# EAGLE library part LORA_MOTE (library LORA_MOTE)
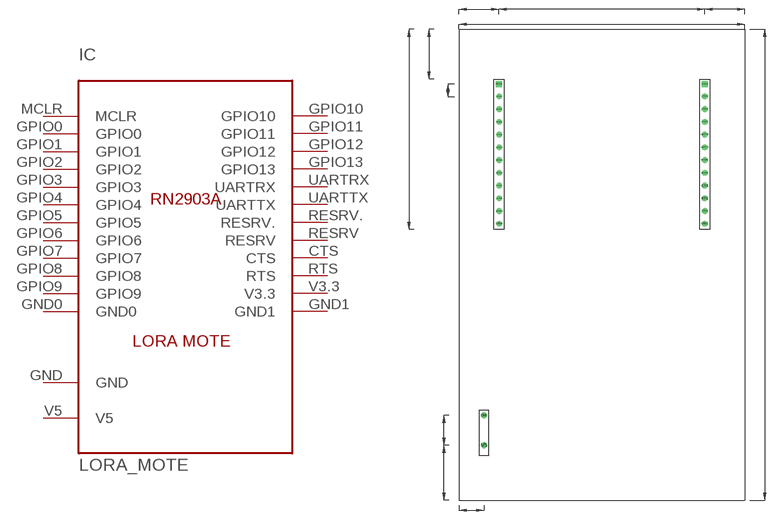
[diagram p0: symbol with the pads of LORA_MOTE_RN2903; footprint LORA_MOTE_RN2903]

Designator prefix IC

## LORA_MOTE  [LORA_MOTE_RN2903]
CTS  CTS
GND  GND
GND0  GND0
GND1  GND1
GPIO0  GPIO0
GPIO1  GPIO1
GPIO2  GPIO2
GPIO3  GPIO3
GPIO4  GPIO4
GPIO5  GPIO5
GPIO6  GPIO6
GPIO7  GPIO7
GPIO8  GPIO8
GPIO9  GPIO9
GPIO10  GPIO10
GPIO11  GPIO11
GPIO12  GPIO12
GPIO13  GPIO13
MCLR  MCLR
RESRV  RESRV
RESRV.  RESRV.
RTS  RTS
UARTRX  UARTRX
UARTTX  UARTTX
V3.3  V3.3
V5  V5

## Footprint LORA_MOTE_RN2903 (pad centres in mm)
drill 0.65: CTS 20.03,8.79; GND -24,-37; GND0 -20.97,1.17; GND1 20.03,1.17; GPIO0 -20.97,26.57; GPIO1 -20.97,24.03; GPIO2 -20.97,21.49; GPIO3 -20.97,18.95; GPIO4 -20.97,16.41; GPIO5 -20.97,13.87; GPIO6 -20.97,11.33; GPIO7 -20.97,8.79; GPIO8 -20.97,6.25; GPIO9 -20.97,3.71; GPIO11 20.03,26.57; GPIO12 20.03,24.03; GPIO13 20.03,21.49; RESRV 20.03,11.33; RESRV. 20.03,13.87; RTS 20.03,6.25; UARTRX 20.03,18.95; UARTTX 20.03,16.41; V3.3 20.03,3.71; V5 -24,-43
drill 0.65 square: GPIO10 20,29; MCLR -21,29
